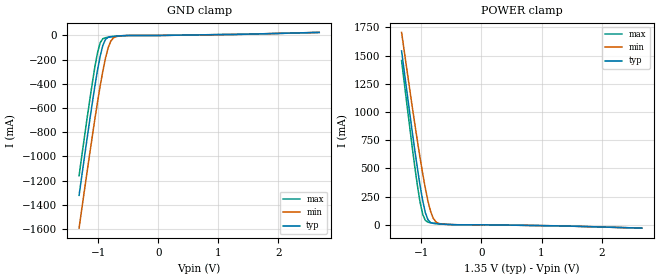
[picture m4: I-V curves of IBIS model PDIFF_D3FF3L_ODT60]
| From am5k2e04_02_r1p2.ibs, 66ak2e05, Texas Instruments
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|   Model PDIFF_D3FF3L_ODT60
[Model] PDIFF_D3FF3L_ODT60
Model_type   Input
Polarity   Non-Inverting
Enable   Active-High
C_comp   3.341pF   3.268pF   3.450pF
C_comp_pullup   618.149fF   582.870fF   680.163fF
C_comp_pulldown 2.716pF   2.679pF   2.764pF
Vinh = 810.000mV
Vinl = 540.000mV
[Temperature Range]   25.000   125.000   -40.000
[Voltage Range]   1.350V   1.283V   1.450V
[GND Clamp Reference]   0.00V   0.00V   0.00V
|[C Comp Corner]
| variable   typ   min   max
|C_comp 3.341pF   3.450pF   3.268pF
|C_comp_pullup 618.149fF   680.163fF   582.870fF
|C_comp_pulldown 2.716pF   2.764pF   2.679pF
[POWER Clamp Reference]   1.350V   1.283V   1.450V
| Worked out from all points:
|   GND clamp passes 1 mA (typ) near -0.55 V on its own axis
|   POWER clamp passes 1 mA (typ) near -0.48 V on its own axis
[GND Clamp]
-1.318V   -1.323A    -1.594A    -1.16A
-1.142V   -706mA     -982.5mA   -539.1mA
-1.055V   -418.4mA   -690.4mA   -259.6mA
-1.011V   -287.1mA   -550.8mA   -142.5mA
-966.7mV  -171.5mA   -418.1mA   -60.49mA
-922.7mV  -82.89mA   -295.5mA   -26.55mA
-878.8mV  -32.7mA    -187.9mA   -18.23mA
-834.9mV  -14.55mA   -103.1mA   -15.08mA
-790.9mV  -9.115mA   -47.58mA   -12.65mA
-747mV    -6.761mA   -19.95mA   -10.39mA
-527.3mV  -543.3uA   -560.9uA   -1.355mA
2.68V     25.6mA     25.47mA    24.97mA
[Power Clamp]
-1.33V    1.541A     1.706A     1.456A
-1.155V   833.7mA    1.055A     696.4mA
-1.067V   503.1mA    744.6mA    349.9mA
-1.023V   351mA      596.1mA    202.1mA
-978.8mV  215.3mA    454.9mA    93.29mA
-934.9mV  108.2mA    324.2mA    39.36mA
-890.9mV  44.09mA    209.7mA    22.55mA
-847mV    19.59mA    118.7mA    17.72mA
-803mV    12.41mA    57.96mA    15mA
-759.1mV  9.598mA    25.89mA    12.62mA
-495.5mV  1.229mA    1.55mA     1.652mA
2.668V    -29.53mA   -29.66mA   -29.81mA
